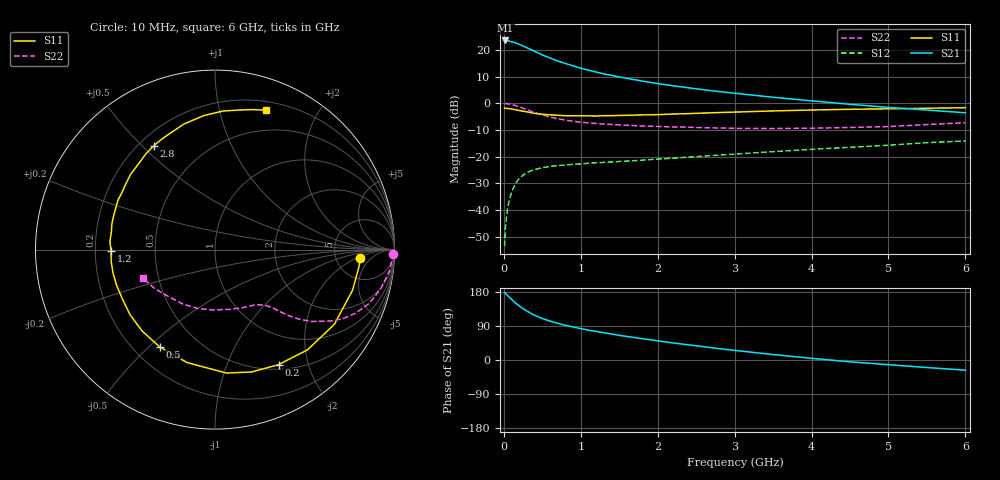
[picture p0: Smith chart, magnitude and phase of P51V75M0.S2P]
! SIEMENS Small Signal Semiconductors
! BFP183
! Si NPN RF Bipolar Junction Transistor in SOT143
! VCE = 1.75 V  IC = 5 mA
! Common Emitter S-Parameters:  March  1996
# GHz  S  MA  R  50
!  f  S11  S21  S12  S22
! GHz  MAG  ANG  MAG  ANG  MAG  ANG  MAG  ANG
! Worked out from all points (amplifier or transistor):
!   36 points, 10 MHz to 6 GHz, reference 50 ohm
!   highest |S21| = 23.6 dB at 20 MHz (marker M1)
!   |S21| within 3 dB of that: start of sweep to 321 MHz
!   unconditionally stable (mu >= 1): 1.531 GHz to 5.768 GHz
!   at 250 MHz: K = 0.21, MSG = 24.2 dB, |S12| = -26.9 dB
!   at 1.4 GHz: K = 0.95, MSG = 16.2 dB, |S12| = -22.0 dB
!   at 6 GHz: K = 0.97, MSG = 5.3 dB, |S12| = -14.1 dB
!   S11 on the Smith chart (normalised r, x): 10 MHz: 8.92, -2.35; 200 MHz: 0.56, -1.55; 500 MHz: 0.30, -0.54; 1.2 GHz: 0.27, -0.00; 2.8 GHz: 0.26, +0.54; 6 GHz: 0.28, +1.40
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0.01  0.8104 -3.2  14.91 178.1  0.0021 86.9  0.9931 -1.3
0.02  0.8083 -6.6  15.08 176.4  0.0046 84.7  0.9884 -2.8
0.05  0.7992 -16.4  14.94 169.8  0.0115 81.7  0.9797 -6.9
0.1  0.7847 -32.0  14.21 160.2  0.0216 72.9  0.9484 -13.5
0.15  0.7598 -47.3  13.64 150.8  0.0311 66.4  0.9086 -19.4
0.2  0.7322 -61.1  12.81 142.6  0.0389 60.3  0.8587 -24.4
0.25  0.7116 -73.4  11.82 135.4  0.045 54.6  0.8084 -28.5
0.3  0.6905 -84.8  11.03 129.2  0.0505 50.4  0.7574 -31.7
0.4  0.6483 -104.0  9.437 118.0  0.0575 43.5  0.6704 -36.7
0.5  0.6235 -119.6  8.055 109.6  0.0619 38.5  0.603 -39.8
0.6  0.6088 -131.9  7.081 102.7  0.0658 35.6  0.5544 -41.7
0.7  0.5962 -142.7  6.207 96.8  0.0679 33.0  0.5152 -43.1
0.9  0.5832 -159.8  5.043 87.2  0.0719 30.7  0.4611 -45.1
1.1  0.5822 -173.4  4.197 78.8  0.0755 29.5  0.4295 -47.0
1.2  0.5795 -179.5  3.858 75.4  0.0768 28.8  0.4197 -48.0
1.7  0.6 156.8  2.766 59.2  0.0843 29.7  0.3814 -54.3
2.2  0.6297 138.5  2.135 45.1  0.0937 30.6  0.3611 -62.3
2.8  0.6718 120.5  1.659 29.9  0.1069 30.5  0.3456 -74.7
3.5  0.7205 104.0  1.299 14.4  0.1243 29.7  0.3367 -91.8
4.5  0.773 86.8  0.958 -4.9  0.1501 25.6  0.3525 -120.7
5.5  0.8079 74.9  0.748 -19.9  0.1829 20.5  0.3998 -146.8
6  0.8278 69.8  0.665 -26.9  0.1975 16.5  0.433 -158.7
